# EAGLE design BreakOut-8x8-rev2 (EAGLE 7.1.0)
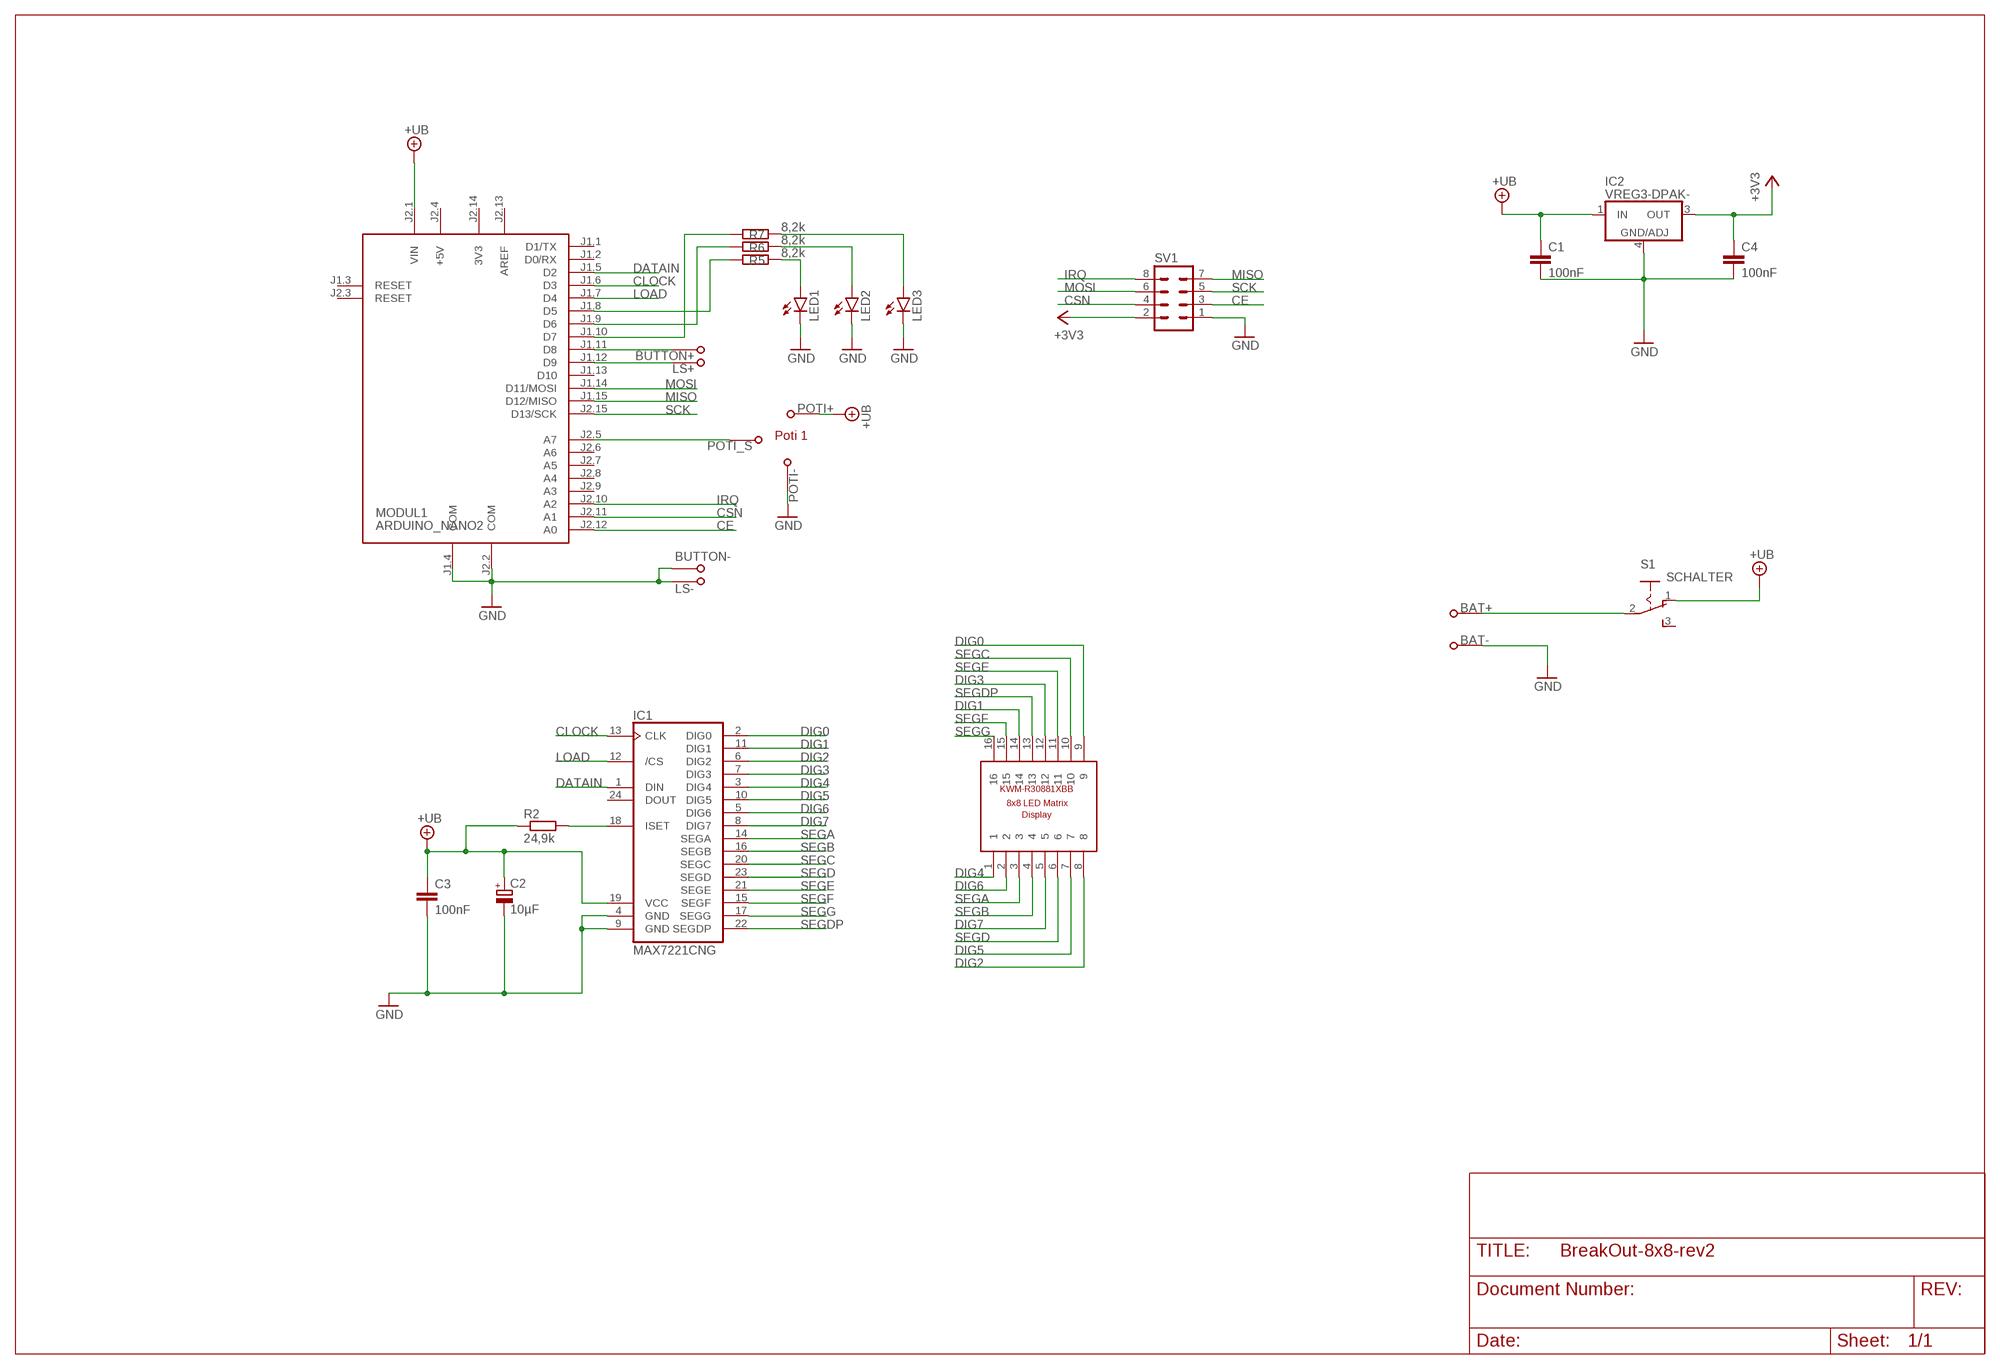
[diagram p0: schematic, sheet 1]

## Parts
BAT+  PAD-NVSMD-2X3  [PAD-SO-2X3]
BAT-  PAD-NVSMD-2X3  [PAD-SO-2X3]
BUTTON+  PAD-NVSMD-2X3  [PAD-SO-2X3]
BUTTON-  PAD-NVSMD-2X3  [PAD-SO-2X3]
C1  100nF  C-EUC0805  [C0805]
C2  10µF  CPOL-EUC/6032-28R  [C/6032-28R]
C3  100nF  C-EUC0805  [C0805]
C4  100nF  C-EUC0805  [C0805]
IC1  MAX7221CNG  [DIL24-3]
IC2  VREG3-DPAK-  [DPAK]
LED1  LED5MM  [LED5MM]
LED2  LED5MM  [LED5MM]
LED3  LED5MM  [LED5MM]
LS+  PAD-NVSMD-2X3  [PAD-SO-2X3]
LS-  PAD-NVSMD-2X3  [PAD-SO-2X3]
MODUL1  ARDUINO_NANO2  [ARDUINO_NANO2]
POTI+  PAD-NVSMD-2X3  [PAD-SO-2X3]
POTI-  PAD-NVSMD-2X3  [PAD-SO-2X3]
POTI_S  PAD-NVSMD-2X3  [PAD-SO-2X3]
R2  24,9k  R-EU_R0805  [R0805]
R5  8,2k  R-EU_R0805  [R0805]
R6  8,2k  R-EU_R0805  [R0805]
R7  8,2k  R-EU_R0805  [R0805]
S1  SCHALTER  [255SB]
SV1  MA04-2  [MA04-2]
U$1  KWM-R30881XBB  [KWM-R30881XBB]

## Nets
+3V3: C4.1 IC2.3(OUT) SV1.2
+UB: C1.1 C2.+ C3.1 IC1.19(VCC) IC2.1(IN) MODUL1.J2.1(VIN) POTI+.1 R2.1 S1.1
BUTTON: MODUL1.J1.10(D7) R7.1
CE: MODUL1.J2.12(A0) SV1.3
CLOCK: IC1.13(CLK) MODUL1.J1.6(D3)
CSN: MODUL1.J2.11(A1) SV1.4
DATAIN: IC1.1(DIN) MODUL1.J1.5(D2)
DIG0: IC1.2(DIG0) U$1.9
DIG1: IC1.11(DIG1) U$1.14
DIG2: IC1.6(DIG2) U$1.8
DIG3: IC1.7(DIG3) U$1.12
DIG4: IC1.3(DIG4) U$1.1
DIG5: IC1.10(DIG5) U$1.7
DIG6: IC1.5(DIG6) U$1.2
DIG7: IC1.8(DIG7) U$1.5
GND: BAT-.1 BUTTON-.1 C1.2 C2.- C3.2 C4.2 IC1.4(GND) IC1.9(GND) IC2.4(GND/ADJ) LED1.K(C) LED2.K(C) LED3.K(C) LS-.1 MODUL1.J1.4(COM) MODUL1.J2.2(COM) POTI-.1 SV1.1
IRQ: MODUL1.J2.10(A2) SV1.8
LOAD: IC1.12(/CS) MODUL1.J1.7(D4)
MISO: MODUL1.J1.15(D12/MISO) SV1.7
MOSI: MODUL1.J1.14(D11/MOSI) SV1.6
N$1: BUTTON+.1 MODUL1.J1.11(D8)
N$2: LED1.A R5.2
N$3: LED2.A R6.2
N$4: LED3.A R7.2
N$5: MODUL1.J2.5(A7) POTI_S.1
N$6: BAT+.1 S1.2
N$17: LS+.1 MODUL1.J1.12(D9)
N$18: IC1.18(ISET) R2.2
N$22: MODUL1.J1.9(D6) R6.1
N$23: MODUL1.J1.8(D5) R5.1
SCK: MODUL1.J2.15(D13/SCK) SV1.5
SEGA: IC1.14(SEGA) U$1.3
SEGB: IC1.16(SEGB) U$1.4
SEGC: IC1.20(SEGC) U$1.10
SEGD: IC1.23(SEGD) U$1.6
SEGDP: IC1.22(SEGDP) U$1.13
SEGE: IC1.21(SEGE) U$1.11
SEGF: IC1.15(SEGF) U$1.15
SEGG: IC1.17(SEGG) U$1.16
Unconnected: IC1.24(DOUT) MODUL1.J1.1(D1/TX) MODUL1.J1.2(D0/RX) MODUL1.J1.3(RESET) MODUL1.J1.13(D10) MODUL1.J2.3(RESET) MODUL1.J2.6(A6) MODUL1.J2.7(A5) MODUL1.J2.8(A4) MODUL1.J2.9(A3) S1.3

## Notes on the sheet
- Poti 1

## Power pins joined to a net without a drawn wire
3V3: MODUL1.J2.14(3V3)
+5V: MODUL1.J2.4(+5V)
AREF: MODUL1.J2.13(AREF)

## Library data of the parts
BAT+ BAT- BUTTON+ BUTTON- LS+ LS- POTI+ POTI- POTI_S = fi-CON:PAD-NV: PAD
C1 C3 C4 = rcl:C-EU: CAPACITOR, European symbol
C2 = rcl:CPOL-EU: POLARIZED CAPACITOR, European symbol
IC1 = maxim-5:MAX7221*: Serially Interfaced, 8-Digit LED Display Drivers
IC2 = sy2002:VREG3-?-*
LED1-LED3 = SparkFun-LED:LED: LEDs
MODUL1 = arduino:ARDUINO_NANO2: Arduino Nano2 Auto generated by modulcreator.ulp \;; ANZAHL: 2; MODUL: TRUE; STECKX0: -76200; STECKX1: 76200; STECKY0: 177800; STECKY1: 177800
R2 R5-R7 = rcl:R-EU_: RESISTOR, European symbol
S1 = sy2002:SCHALTER
SV1 = con-lstb:MA04-2: PIN HEADER; OC_FARNELL: unknown; OC_NEWARK: unknown
U$1 = sy2002:KWM-R30881XBB: 8x8 LED Matrix Display KWM-R30881ABB KWM-R30881CBB

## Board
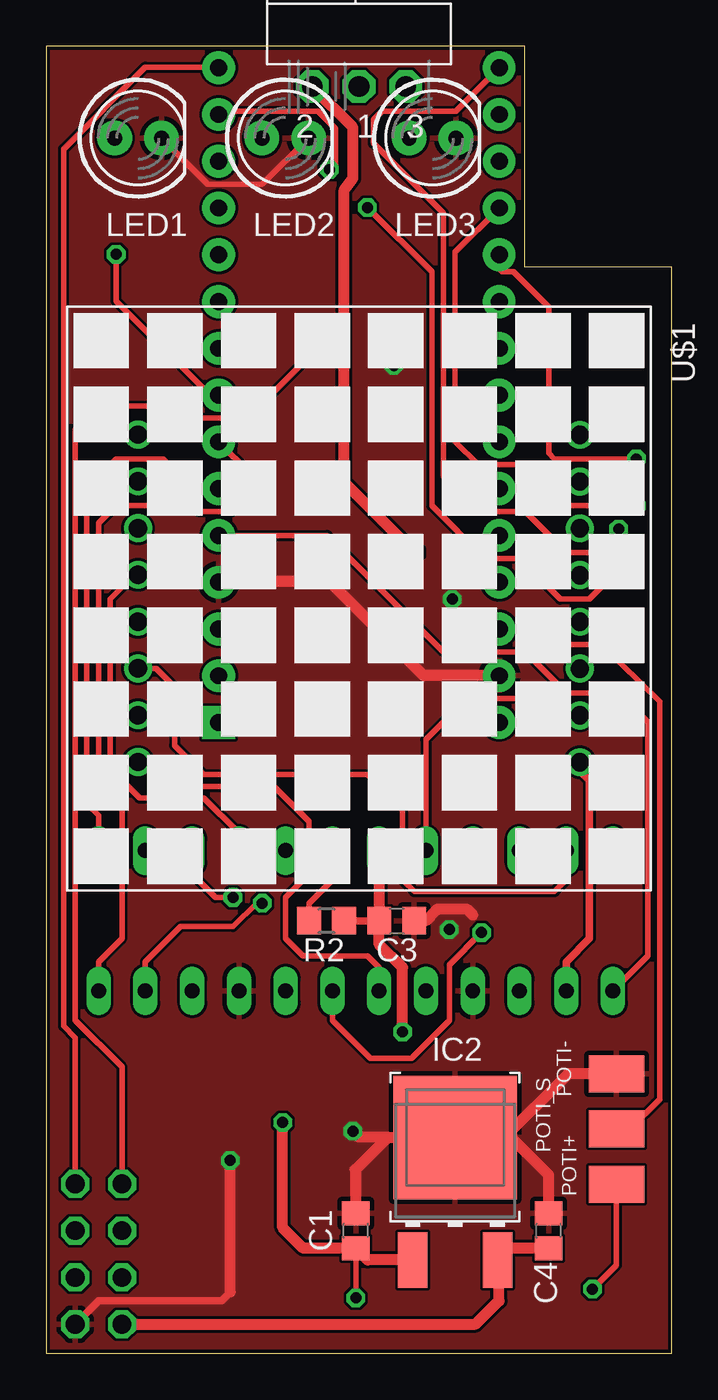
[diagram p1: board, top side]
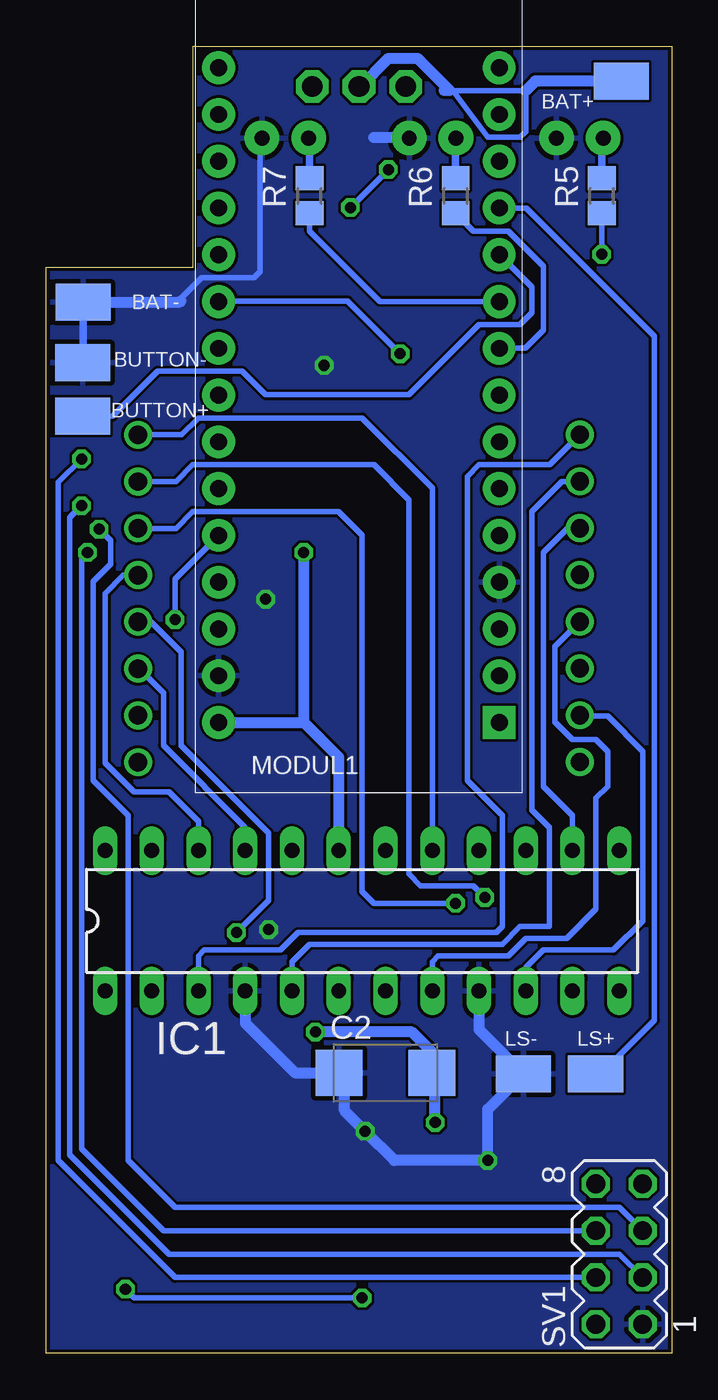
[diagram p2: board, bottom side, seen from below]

Size 34 x 71 mm. Coordinates in mm from the lower left corner, seen from the top.
Outline: 0,0 34,0 34,59 26,59 26,71 0,71 0,0
Copper layers (1*16): Top 0.035mm / dielectric 1.5mm / Bottom 0.035mm
Design rules "default *": minimum track width 10mil, minimum drill 12mil, track to track 6mil, track to pad 6mil, pad to pad 6mil, via to via 6mil, smd to smd 6mil, copper to edge 8mil, drill to drill 8mil, minimum pad ring 10mil, minimum via ring 8mil, stop-mask expansion 4mil, vias tented up to drill 0mil, thermal gap 10mil

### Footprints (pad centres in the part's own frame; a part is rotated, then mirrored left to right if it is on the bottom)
PAD-SO-2X3 = smd 3 x 2: 1 0,0
C0805 = smd 1.3 x 1.5: 1 -0.95,0; 2 0.95,0
C/6032-28R = smd 2.55 x 2.5: + 2.525,0; - -2.525,0
DIL24-3 = drill 0.813 long: 1 -13.97,-3.81; 2 -11.43,-3.81; 3 -8.89,-3.81; 4 -6.35,-3.81; 5 -3.81,-3.81; 6 -1.27,-3.81; 7 1.27,-3.81; 8 3.81,-3.81; 9 6.35,-3.81; 10 8.89,-3.81; 11 11.43,-3.81; 12 13.97,-3.81; 13 13.97,3.81; 14 11.43,3.81; 15 8.89,3.81; 16 6.35,3.81; 17 3.81,3.81; 18 1.27,3.81; 19 -1.27,3.81; 20 -3.81,3.81; 21 -6.35,3.81; 22 -8.89,3.81; 23 -11.43,3.81; 24 -13.97,3.81
DPAK = smd 1.6 x 3: 1 -2.3,0; 3 2.3,0 | smd 6.7 x 6.7: 4 0,6.65
LED5MM = drill 0.813 pad 1.88: A -1.27,0; K 1.27,0
ARDUINO_NANO2 = drill 0.914 pad 1.778 square: J1.1 -7.62,17.78 | drill 0.914 pad 1.778: J1.2 -7.62,15.24; J1.3 -7.62,12.7; J1.4 -7.62,10.16; J1.5 -7.62,7.62; J1.6 -7.62,5.08; J1.7 -7.62,2.54; J1.8 -7.62,0; J1.9 -7.62,-2.54; J1.10 -7.62,-5.08; J1.11 -7.62,-7.62; J1.12 -7.62,-10.16; J1.13 -7.62,-12.7; J1.14 -7.62,-15.24; J1.15 -7.62,-17.78; J2.1 7.62,17.78; J2.2 7.62,15.24; J2.3 7.62,12.7; J2.4 7.62,10.16; J2.5 7.62,7.62; J2.6 7.62,5.08; J2.7 7.62,2.54; J2.8 7.62,0; J2.9 7.62,-2.54; J2.10 7.62,-5.08; J2.11 7.62,-7.62; J2.12 7.62,-10.16; J2.13 7.62,-12.7; J2.14 7.62,-15.24; J2.15 7.62,-17.78
R0805 = smd 1.3 x 1.5: 1 -0.95,0; 2 0.95,0
255SB = drill 1.118 pad 1.778 octagon: 1 -2.54,0; 2 0,0; 3 2.54,0
MA04-2 = drill 1.016 octagon: 1 -3.81,-1.27; 2 -3.81,1.27; 3 -1.27,-1.27; 4 -1.27,1.27; 5 1.27,-1.27; 6 1.27,1.27; 7 3.81,-1.27; 8 3.81,1.27
KWM-R30881XBB = drill 1: 1 -8.9,-12; 2 -6.36,-12; 3 -3.82,-12; 4 -1.28,-12; 5 1.26,-12; 6 3.8,-12; 7 6.34,-12; 8 8.88,-12; 9 8.89,12; 10 6.35,12; 11 3.81,12; 12 1.27,12; 13 -1.27,12; 14 -3.81,12; 15 -6.35,12; 16 -8.89,12

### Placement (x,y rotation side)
BAT+  2.75,69.09 0 bottom
BAT-  31.98,57.09 0 bottom
BUTTON+  32.01,50.9 0 bottom
BUTTON-  32.01,53.81 0 bottom
C1  16.83,6.67 90 top
C2  15.56,15.24 0 bottom
C3  19.05,23.5 0 top
C4  27.3,6.67 90 top
IC1  16.83,23.5 0 bottom
IC2  22.23,5.08 0 top
LED1  5,66 0 top
LED2  13,66 0 top
LED3  21,66 0 top
LS+  4.15,15.19 0 bottom
LS-  8.07,15.19 0 bottom
MODUL1  17,52.05 180 bottom
POTI+  30.99,9.19 0 top
POTI-  30.99,15.19 0 top
POTI_S  30.99,12.19 0 top
R2  15.24,23.5 180 top
R5  3.81,62.87 90 bottom
R6  11.75,62.87 90 bottom
R7  19.68,62.87 90 bottom
S1  17,68.8 0 top
SV1  2.86,5.4 90 bottom
U$1  17,41 270 top

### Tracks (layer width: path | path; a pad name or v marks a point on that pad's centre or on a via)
+3V3
  Top 0.61: SV1.2 23.34,1.59 24.61,2.86 24.61,5 IC2.3 25.16,5.72 C4.1
+UB  (via drill 0.6)
  Top 0.305: POTI+.1 30.99,4.8 v29.69,3.49 | v16.83,3.02 C1.1
  Top 0.406: R2.1 C3.1
  Top 0.61: IC1.19 C3.1 18.1,22.23 19.37,20.95 v19.37,17.46 | IC2.1 17.46,5.08 C1.1 13.97,5.72 12.86,6.83 v12.86,12.54 | v20,43.5 16.19,47.31 16.19,63.18 16.67,63.82 16.67,66.59 S1.1
  Bottom 0.305: v29.69,3.49 29.21,3.02 v16.83,3.02
  Bottom 0.61: MODUL1.J2.1 19.98,34.27 | 19.98,34.27 18.1,32.38 IC1.19 | v19.37,17.46 14.13,17.46 13.03,16.37 C2.+ 12.86,15.07 v12.86,12.54 | 19.98,34.27 19.98,43.47 v20,43.5
BUTTON
  Bottom 0.305: MODUL1.J1.10 15.85,57.12 19.68,60.96 R7.1
CE  (via drill 0.6)
  Top 0.305: v32.07,46.04 28.26,46.04 26.04,48.26 23.5,48.26 22.23,49.53 22.23,59.81 MODUL1.J2.12
  Bottom 0.305: SV1.3 2.86,5.4 27.3,5.4 32.7,10.79 32.7,45.4 v32.07,46.04
CLOCK
  Top 0.305: MODUL1.J1.6 7.96,46.97 6.35,48.58 3.81,48.58 2.22,46.99 2.22,29.84 2.86,29.21 IC1.13
CSN  (via drill 0.6)
  Top 0.305: v32.07,48.58 27.62,48.58 27.3,48.9 27.3,56.83 25.4,58.74 24.77,58.74 24.45,59.05 24.45,59.49 MODUL1.J2.11
  Bottom 0.305: SV1.4 26.99,4.13 33.34,10.48 33.34,47.31 v32.07,48.58
DATAIN
  Top 0.305: MODUL1.J1.5 15.27,44.42 21.59,38.1 26.04,38.1 28.26,35.88 31.11,35.88 32.7,34.29 32.7,21.59 IC1.1
DIG0
  Top 0.406: U$1.9 29,31.64 29.53,31.11 29.53,22.54 28.26,21.27 IC1.2
DIG1  (via drill 0.6)
  Top 0.305: v11.75,24.45 11.43,24.45 10.16,23.18 7.3,23.18 5.4,21.27 IC1.11
  Bottom 0.305: U$1.14 26.95,44.81 26.04,45.72 18.1,45.72 16.83,44.45 16.83,25.08 16.19,24.45 v11.75,24.45
DIG2
  Top 0.305: U$1.8 6.3,32.12 7.62,30.8 12.38,30.8 14.29,28.89 14.29,26.04 13.02,24.77 13.02,22.54 13.97,21.59 17.46,21.59 18.1,20.95 IC1.6
DIG3  (via drill 0.6)
  Top 0.305: v23.65,22.86 21.91,21.11 21.91,18.1 19.84,16.03 17.62,16.03 15.56,18.1 IC1.7
  Bottom 0.305: U$1.12 28.3,39.73 26.67,38.1 26.67,33.02 21.91,28.26 21.91,24.61 v23.65,22.86
DIG4
  Bottom 0.305: IC1.3 25.72,21.59 25.4,21.91 21.27,21.91 20.32,22.86 9.53,22.86 9.21,23.18 9.21,29.21 11.11,31.11 11.11,47.62 10.48,48.26 6.64,48.26 U$1.1
DIG5
  Bottom 0.305: IC1.10 7.94,20.95 6.99,21.91 3.17,21.91 1.59,23.5 1.59,32.7 3.49,34.61 4.95,34.61 U$1.7
DIG6
  Bottom 0.305: U$1.2 5.98,47.36 7.62,45.72 7.62,29.53 6.67,28.57 6.67,23.18 8.26,23.18 9.21,22.23 19.68,22.23 20.64,21.27 IC1.5
DIG7
  Bottom 0.305: IC1.8 13.02,21.27 12.7,21.59 8.89,21.59 7.94,22.54 5.71,22.54 4.13,24.13 4.13,30.16 3.49,30.8 3.49,32.7 4.13,33.34 5.4,33.34 6.35,34.29 6.35,38.39 U$1.5
GND  (via drill 0.6)
  Top 0.305: LED2.K 14.25,66 11.75,63.5 8.77,63.5 LED1.K
  Top 0.406: SV1.1 2.86,2.86 9.53,2.86 10,3.33 | 16.67,10 16.83,9.84
  Top 0.61: C3.2 20.64,23.5 21.27,24.13 22.86,24.13 23.18,23.81 | MODUL1.J2.2 20.5,36.8 15.4,41.91 9.4,41.91 MODUL1.J1.4 | C4.2 27.3,9.68 25.4,11.59 24.77,11.59 | 24.77,11.59 22.37,11.59 IC2.4 22.21,11.75 18.57,11.75 | POTI-.1 28.37,15.19 24.77,11.59 | C1.2 16.83,9.84 16.83,10 18.57,11.75 | 18.57,11.75 16.99,11.75 v16.67,12.06 | 10,3.33 v10,10.48
  Bottom 0.305: 26.67,57.15 26.67,57.31 25.56,58.42 22.7,58.42 22.38,58.74 22.38,65.89 LED3.K
  Bottom 0.406: BAT-.1 31.98,53.84 BUTTON-.1
  Bottom 0.61: LED3.K 22.27,66.15 | 16.19,66.04 14.31,66.04 LED2.K | BAT-.1 26.73,57.09 26.67,57.15 | IC1.4 23.18,17.94 20.48,15.24 C2.- 17.78,14.94 17.78,13.18 v16.67,12.06 15.08,10.48 v10,10.48 10,13.26 LS-.1 10.48,17.6 IC1.9
  other vias: 18.89,53.66 22.07,40.96 21.91,23.02
  pour Bottom: 0,0 33.81,0 33.81,70.8 0,70.8
  pour Top: 0,0 33.97,0 33.97,70.96 0,70.96
IRQ  (via drill 0.6)
  Top 0.305: SV1.8 4.13,15.56 1.59,18.1 1.59,50.16 2.86,51.44 7.62,51.44 8.26,50.8 10.95,50.8 14.45,54.29 v14.76,54.29
  Bottom 0.305: v14.76,54.29 17.62,57.15 24.59,57.15 MODUL1.J2.10
LOAD
  Top 0.305: IC1.12 2.86,21.27 4.13,22.54 4.13,30.16 2.86,31.43 2.86,45.09 3.81,46.04 7.94,46.04 8.26,45.72 10.16,45.72 11.11,46.67 11.11,47.77 MODUL1.J1.7
MISO
  Top 0.305: SV1.7 1.59,17.14 0.95,17.78 0.95,65.41 5.4,69.85 9.36,69.85 MODUL1.J1.15
MOSI  (via drill 0.6)
  Top 0.305: v31.75,43.5 31.75,43.18 29.53,40.96 27.94,40.96 25.72,43.18 23.81,43.18 20.95,46.04 20.95,58.74 v17.46,62.23 | MODUL1.J1.14 9.88,67.47 14.76,67.47 15.72,66.52 15.72,64.61 v15.4,64.29
  Bottom 0.305: SV1.6 27.62,6.67 32.07,11.11 32.07,43.18 v31.75,43.5 | v17.46,62.23 v15.4,64.29
N$1
  Bottom 0.305: BUTTON+.1 30.39,50.9 27.94,53.34 23.34,53.34 22.07,52.07 14.29,52.07 10.48,55.88 8.26,55.88 7.62,56.52 7.62,57.91 MODUL1.J1.11
N$2
  Bottom 0.406: R5.2 3.81,65.92 LED1.A
N$3
  Bottom 0.406: R6.2 11.75,65.98 LED2.A
N$4
  Bottom 0.406: R7.2 19.68,65.95 LED3.A
N$5  (via drill 0.6)
  Top 0.305: POTI_S.1 31.72,12.19 33.34,13.81 33.34,35.4 30.16,38.5 28.26,38.5 v26.99,39.85
  Bottom 0.305: v26.99,39.85 26.99,42.06 MODUL1.J2.5
N$6
  Bottom 0.305: 11.91,68.58 7.94,68.58 7.94,66.36 8.26,66.04 10,66.04 11.91,68.58 | 11.91,68.58 12.06,68.58
  Bottom 0.61: BAT+.1 7.42,69.09 7.94,68.58 | 12.38,68.58 12.06,68.58 13.81,70.33 15.4,70.33 16.93,68.8 S1.2
N$17
  Bottom 0.305: LS+.1 3.86,15.19 0.95,18.1 0.95,55.24 7.91,62.2 MODUL1.J1.12
N$18
  Top 0.305: IC1.18 15.56,25.72 14.29,24.45 R2.2
N$22
  Bottom 0.305: MODUL1.J1.9 7.96,54.59 6.99,55.56 6.99,59.05 8.89,60.96 10.79,60.96 R6.1
N$23  (via drill 0.6)
  Top 0.305: MODUL1.J1.8 8.91,52.05 3.81,57.15 v3.81,59.69
  Bottom 0.305: v3.81,59.69 R5.1
SCK  (via drill 0.6)
  Top 0.305: v31.11,44.77 29.84,43.5 28.26,43.5 26.04,45.72 23.5,45.72 21.59,47.62 21.59,61.91 17.78,65.72 17.78,66.99 18.26,67.47 22.26,67.47 MODUL1.J2.15
  Bottom 0.305: SV1.5 2.86,7.94 26.99,7.94 29.53,10.48 29.53,29.21 31.43,31.11 31.43,41.91 30.48,42.86 30.48,44.13 v31.11,44.77
SEGA
  Bottom 0.305: U$1.3 5.66,44.82 6.99,43.5 6.99,30.8 5.4,29.21 IC1.14
SEGB
  Top 0.305: U$1.4 4.82,42.28 3.49,40.96 3.49,31.75 5.08,30.16 8.57,30.16 10.48,28.26 IC1.16
SEGC
  Top 0.305: U$1.10 27.58,34.65 26.67,35.56 22.86,35.56 20.64,33.34 IC1.20
SEGD
  Top 0.305: U$1.6 5.98,37.2 6.99,36.2 6.99,33.02 8.57,31.43 17.46,31.43 19.37,29.53 19.37,25.72 20,25.08 27.62,25.08 28.26,25.72 IC1.23
SEGDP
  Bottom 0.305: U$1.13 29.8,42.27 30.8,41.27 30.8,32.07 29.21,30.48 27.3,30.48 25.72,28.89 IC1.22
SEGE
  Bottom 0.305: U$1.11 28.93,37.19 27.62,35.88 27.62,33.02 23.18,28.57 IC1.21
SEGF  (via drill 0.6)
  Top 0.305: v10.16,24.77 9.21,24.77 7.94,26.04 IC1.15
  Bottom 0.305: U$1.15 26.95,47.35 26.04,48.26 16.19,48.26 14.29,46.35 14.29,26.04 13.65,25.4 10.79,25.4 v10.16,24.77
SEGG
  Bottom 0.305: U$1.16 26.63,49.89 25.72,50.8 16.83,50.8 13.02,46.99 IC1.17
